// ------------------------------------------------------------------
// File           : D:\PRESETTTT.awl
//
// Source File    : D:\PRESET.var
// Generation Date: 9/13/2017  Time: 6:31:10 PM
// ------------------------------------------------------------------

DATA_BLOCK DB  120
VERSION : 0.0


STRUCT

 C1_SEMA_PRESETVal3_4:
   STRUCT
   SYNTAX_ID : BYTE := B#16#82;
   bereich_u_einheit : BYTE := B#16#41;
   spalte : WORD := W#16#4;
   zeile : WORD := W#16#3;
   bausteintyp : BYTE := B#16#71;
   ZEILENANZAHL : BYTE := B#16#1;
   typ : BYTE := B#16#F;
   laenge : BYTE := B#16#8;
   END_STRUCT ;

 END_STRUCT ;

BEGIN
END_DATA_BLOCK
